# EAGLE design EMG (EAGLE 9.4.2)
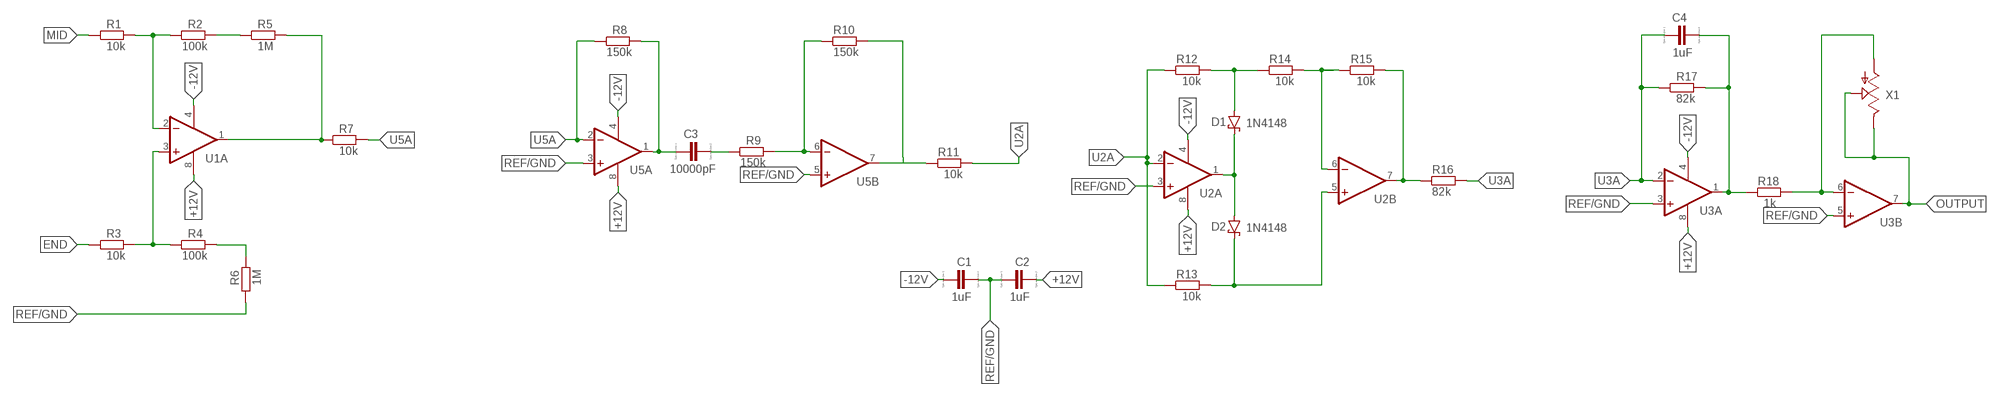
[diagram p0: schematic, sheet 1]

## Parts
C1  1uF  SURFACEMOUNTCC1310  [C1310]
C2  1uF  SURFACEMOUNTCC1310  [C1310]
C3  10000pF  SURFACEMOUNTCC1310  [C1310]
C4  1uF  SURFACEMOUNTCC1310  [C1310]
D1  1N4148  SURFACEMOUNTDIODE  [SOD323_ST]
D2  1N4148  SURFACEMOUNTDIODE  [SOD323_ST]
R1  10k  RESISTORSM0805  [SURFACEMOUNT]
R2  100k  RESISTORSM0805  [SURFACEMOUNT]
R3  10k  RESISTORSM0805  [SURFACEMOUNT]
R4  100k  RESISTORSM0805  [SURFACEMOUNT]
R5  1M  RESISTORSM0805  [SURFACEMOUNT]
R6  1M  RESISTORSM0805  [SURFACEMOUNT]
R7  10k  RESISTORSM0805  [SURFACEMOUNT]
R8  150k  RESISTORSM0805  [SURFACEMOUNT]
R9  150k  RESISTORSM0805  [SURFACEMOUNT]
R10  150k  RESISTORSM0805  [SURFACEMOUNT]
R11  10k  RESISTORSM0805  [SURFACEMOUNT]
R12  10k  RESISTORSM0805  [SURFACEMOUNT]
R13  10k  RESISTORSM0805  [SURFACEMOUNT]
R14  10k  RESISTORSM0805  [SURFACEMOUNT]
R15  10k  RESISTORSM0805  [SURFACEMOUNT]
R16  82k  RESISTORSM0805  [SURFACEMOUNT]
R17  82k  RESISTORSM0805  [SURFACEMOUNT]
R18  1k  RESISTORSM0805  [SURFACEMOUNT]
U1  OPAMPSUA  [SOIC8]
U2  OPAMPSUA  [SOIC8]
U3  OPAMPSUA  [SOIC8]
U5  OPAMPSUA  [SOIC8]
X1  POTENTIOMETERS3223G  [SURFACEMOUNTPOT]

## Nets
+12V: C2.2 U1.8(P:V+) U2.8(P:V+) U3.8(P:V+) U5.8(P:V+)
-12V: C1.1 U1.4(P:V-) U2.4(P:V-) U3.4(P:V-) U5.4(P:V-)
END: R3.1
MID: R1.1
N$1: R1.2 R2.1 U1.2(A:-IN)
N$2: R3.2 R4.1 U1.3(A:+IN)
N$3: R2.2 R5.1
N$4: R4.2 R6.2
N$5: R15.2 R16.1 U2.7(B:OUT)
N$6: C3.1 R8.2 U5.1(A:OUT)
N$7: C3.2 R9.1
N$8: R9.2 R10.1 U5.6(B:-IN)
N$9: R18.2 U3.6(B:-IN) X1.1(A)
N$10: R14.2 R15.1 U2.6(B:-IN)
N$11: D1.C D2.A U2.1(A:OUT)
N$12: D1.A R12.2 R14.1
N$13: D2.C R13.2 U2.5(B:+IN)
N$14: C4.2 R17.2 R18.1 U3.1(A:OUT)
N$15: R10.2 R11.1 U5.7(B:OUT)
N$17: R5.2 R7.1 U1.1(A:OUT)
OUTPUT: U3.7(B:OUT) X1.2(S) X1.3(E)
REF/GND: C1.2 C2.1 R6.1 U2.3(A:+IN) U3.3(A:+IN) U3.5(B:+IN) U5.3(A:+IN) U5.5(B:+IN)
U2A: R11.2 R12.1 R13.1 U2.2(A:-IN)
U3A: C4.1 R16.2 R17.1 U3.2(A:-IN)
U5A: R7.2 R8.1 U5.2(A:-IN)
Unconnected: U1.5(B:+IN) U1.6(B:-IN) U1.7(B:OUT)

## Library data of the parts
C1-C4 = Customized:SURFACEMOUNTC: CAPACITOR, European symbol; SPICEMODEL: NONE; SPICEPREFIX: C
D1 D2 = Customized:SURFACEMOUNTDIODE: Schottky barrier diode
R1-R18 = Customized:RESISTORS: RESISTOR, European symbol; SPICEPREFIX: R
U1-U3 U5 = Customized:OPAMPS: 12V, 7MHz, CMOS, Rail-to-Rail I/O Dual OP AMP Source: http://focus.ti.com/lit/ds/sbos201/sbos201.pdf
X1 = Customized:POTENTIOMETERS: POTENTIOMETER

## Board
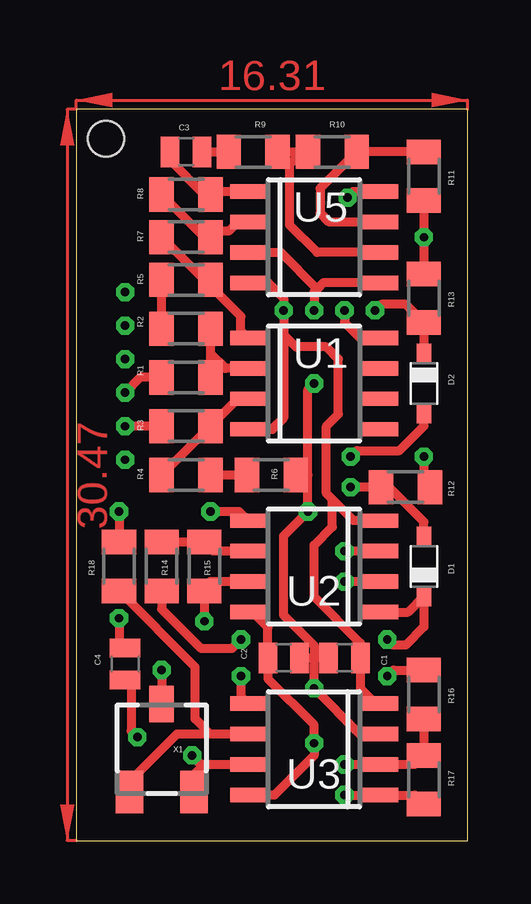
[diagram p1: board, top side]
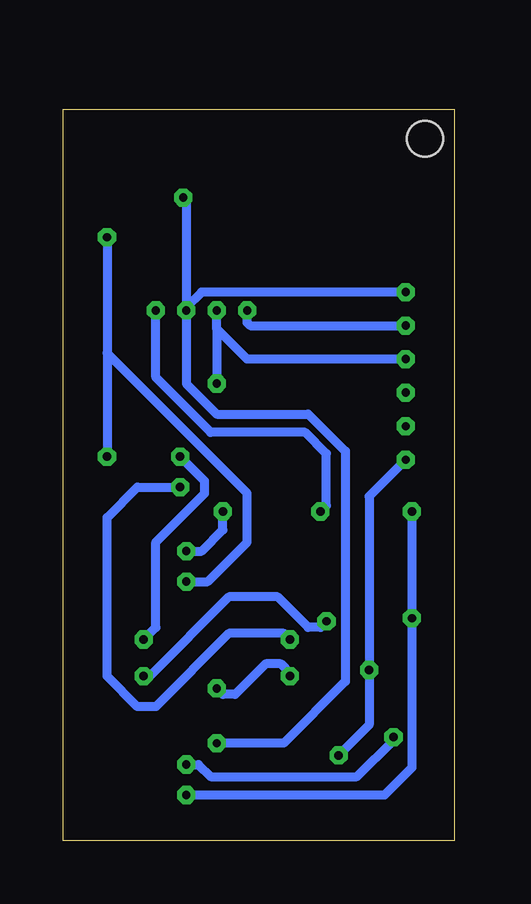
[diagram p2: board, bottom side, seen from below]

Size 16.31 x 30.47 mm. Coordinates in mm from the lower left corner, seen from the top.
Outline: 0,0 16.31,0 16.31,30.47 0,30.47 0,0
Copper layers (1*16): Top 0.035mm / dielectric 1.5mm / Bottom 0.035mm
Design rules "default": minimum track width 6mil, minimum drill 0.35mm, track to track 6mil, track to pad 6mil, pad to pad 6mil, via to via 6mil, smd to smd 6mil, copper to edge 40mil, drill to drill 6mil, minimum pad ring 10mil, minimum via ring 8mil, stop-mask expansion 4mil, vias tented up to drill 0mil, thermal gap 10mil
Holes 1.5 mm at 1.23,29.25

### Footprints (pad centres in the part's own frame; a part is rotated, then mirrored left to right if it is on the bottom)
C1310 = smd 0.771 x 1.27: 1 -0.66,0; 2 0.66,0
SOD323_ST = smd 0.8 x 0.6: A 1.25,0; C -1.25,0
SURFACEMOUNT = smd 1.016 x 1.422: 1 -1.016,0; 2 1.016,0
SOIC8 = smd 0.6 x 1.5: 1 -1.905,-2.75; 2 -0.635,-2.75; 3 0.635,-2.75; 4 1.905,-2.75; 5 1.905,2.75; 6 0.635,2.75; 7 -0.635,2.75; 8 -1.905,2.75
SURFACEMOUNTPOT = smd 1.143 x 1.778: 1 -1.346,-1.778; 3 1.346,-1.778 | smd 1.016 x 1.524: 2 0,1.88

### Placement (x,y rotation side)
C1  11.18,7.62 180 top
C2  8.64,7.62 180 top
C3  4.57,28.7 0 top
C4  2.03,7.37 90 top
D1  14.48,11.43 90 top
D2  14.48,19.05 270 top
R1  4.57,19.3 0 top
R2  4.57,21.34 180 top
R3  4.57,17.27 0 top
R4  4.57,15.24 0 top
R5  4.57,23.37 0 top
R6  8.13,15.24 180 top
R7  4.57,25.15 0 top
R8  4.57,26.92 0 top
R9  7.37,28.7 0 top
R10  10.67,28.7 0 top
R11  14.48,27.69 270 top
R12  13.72,14.73 180 top
R13  14.48,22.61 270 top
R14  3.56,11.43 90 top
R15  5.33,11.43 270 top
R16  14.48,6.1 270 top
R17  14.48,2.54 270 top
R18  1.78,11.43 270 top
U1  9.91,19.05 270 top
U2  9.91,11.43 90 top
U3  9.91,3.81 90 top
U5  9.91,25.15 270 top
X1  3.56,3.81 0 top

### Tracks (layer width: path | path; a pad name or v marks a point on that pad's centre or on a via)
+12V  (via drill 0.35 pad 0.38)
  Top 0.381: U1.8 11.81,20.95 11.18,21.59 v11.18,22.1 | U2.8 7.34,9.53 7.98,8.89 C2.2 7.98,6.76 9.91,4.83 v9.91,4.06 9.91,3.56 8.26,1.91 U3.8 | U5.8 11.56,27.05 v11.3,26.8
  Bottom 0.381: v2.03,22.86 10.54,22.86 11.18,22.23 | v11.3,26.8 11.18,26.67 11.18,22.23 | v9.91,4.06 7.12,4.06 4.55,6.64 4.55,16.23 6.1,17.78 9.91,17.78 11.18,19.05 v11.18,22.1 11.18,22.23
-12V  (via drill 0.35 pad 0.38)
  Top 0.381: U1.4 8.17,17.14 8.64,17.61 8.64,21.08 | U3.4 12.47,5.71 11.84,6.35 C1.1 11.84,8.23 9.91,10.16 9.91,12.32 10.67,13.08 10.67,14.22 | U5.4 8,23.24 8.64,22.61 v8.64,22.1 8.64,21.08 | 8.64,21.08 9.14,20.57 10.41,20.57 10.92,20.07 10.92,17.78 10.41,17.27 10.41,14.48 10.67,14.22 | U2.4 11.56,13.34 10.67,14.22
  Bottom 0.381: v8.64,22.1 8.64,21.59 8.51,21.46 v2.03,21.46
END  (via drill 0.35 pad 0.38)
  Top 0.381: R3.1 v2.03,17.27
MID  (via drill 0.35 pad 0.38)
  Top 0.381: R1.1 2.67,19.3 v2.03,18.67
N$1
  Top 0.381: 5.97,19.68 U1.2 6.22,19.68 5.59,20.32 | R2.1 5.59,20.32 | 5.59,20.32 R1.2
N$2
  Top 0.381: U1.3 6.73,18.41 R3.2 R4.1
N$3
  Top 0.381: R2.2 R5.1
N$4
  Top 0.381: R4.2 R6.2
N$5  (via drill 0.35 pad 0.38)
  Top 0.381: v5.33,9.14 R15.2 5.33,10.54 5.59,10.79 U2.7 | R16.1 13.21,7.11 v12.95,6.86
  Bottom 0.381: v12.95,6.86 12.7,6.86 9.4,10.16 7.37,10.16 6.1,8.89 5.59,8.89 v5.33,9.14
N$6
  Top 0.381: 7.09,27.05 U5.1 5.71,27.05 R8.2 5.33,26.92 3.91,28.35 C3.1
N$7
  Top 0.381: C3.2 R9.1
N$8
  Top 0.381: 8.64,28.7 R9.2 9.4,28.7 | 9.4,28.7 R10.1 | U5.6 10.03,24.51 8.89,25.65 8.89,28.19 9.4,28.7
N$9
  Top 0.381: X1.1 2.21,2.46 4.19,4.45 U3.6 5.59,4.45 4.95,5.08 4.95,7.24 R18.2
N$10
  Top 0.381: 3.58,12.72 R14.2 R15.1 5.71,12.06 U2.6
N$11  (via drill 0.35, 0.35 pad 0.33)
  Top 0.381: 11.61,16.18 v11.43,16 11.68,16.26 13.46,16.26 14.48,17.27 D2.A | 12.91,9.53 U2.1 13.82,9.53 D1.C 14.48,8.91 13.72,8.15 13.19,8.15 v12.95,8.38
  Bottom 0.381: v11.43,16 10.41,14.99 10.41,14.48 12.45,12.45 12.45,8.89 v12.95,8.38
N$12  (via drill 0.35 pad 0.33, 0.35 pad 0.38)
  Top 0.381: 6.83,8.38 v6.86,8.38 6.48,8 5.21,8 3.56,9.65 R14.1 | R12.2 12.7,14.88 | R12.2 v11.43,14.73 | 13.03,14.73 R12.2 | 12.79,14.73 R12.2 | D1.A 14.48,13.28 13.03,14.73 R12.2
  Bottom 0.381: v11.43,14.73 13.21,14.73 14.48,13.46 14.48,6.86 13.21,5.59 12.45,5.59 9.4,8.64 7.11,8.64 v6.86,8.38
N$13  (via drill 0.35, 0.35 pad 0.38)
  Top 0.381: U2.5 6.78,13.72 v5.59,13.72 | v12.45,22.1 12.7,22.35 13.72,22.35 R13.2 D2.C
  Bottom 0.381: v12.45,22.1 12.45,19.3 10.16,17.02 6.22,17.02 5.33,16.13 5.33,13.97 v5.59,13.72
N$14  (via drill 0.35, 0.35 pad 0.33)
  Top 0.381: U3.1 13.08,1.91 | v1.78,13.72 R18.1 | v11.18,1.91 U3.1 | U3.1 14.1,1.91 R17.2 | v1.78,9.27 1.78,8.28 C4.2
  Bottom 0.381: v1.78,13.72 v1.78,9.27 1.78,3.05 2.92,1.91 v11.18,1.91
N$15
  Top 0.381: 14.22,28.7 R11.1 R10.2 10.16,27.18 10.16,26.16 10.54,25.78 U5.7
N$17
  Top 0.381: 5.33,23.37 R7.1 | 5.33,23.37 R5.2 5.59,23.11 | U1.1 6.86,21.25 6.86,21.84 5.33,23.37
OUTPUT  (via drill 0.35, 0.35 pad 0.38)
  Top 0.381: v3.56,7.11 X1.2 | U3.7 5.33,3.17 | 5.33,3.17 5.21,3.17 v4.83,3.56 | X1.3 4.9,2.74 5.33,3.17
  Bottom 0.381: v2.03,15.88 3.56,14.35 v3.56,7.11 3.56,4.83 v4.83,3.56
REF/GND  (via drill 0.35, 0.35 pad 0.33, 0.35 pad 0.38)
  Top 0.381: C2.1 9.93,7.62 | C1.2 9.93,7.62 | 9.93,7.62 9.93,8.1 8.64,9.4 8.64,12.7 v9.65,13.72 9.65,15.24 | 12.57,12.06 U2.3 v11.18,12.06 | U3.5 6.86,6.01 v6.86,6.86 | v9.91,19.05 9.65,18.8 9.65,15.24 | R6.1 9.65,15.24 | U5.3 8.51,24.51 10.03,22.99 | v9.91,22.1 9.91,22.86 10.03,22.99 | U5.5 10.29,23.24 10.03,22.99 | 9.93,7.62 9.91,7.59 v9.91,6.35 11.81,4.45 U3.3
  Bottom 0.381: v11.18,12.06 10.54,12.06 9.65,12.95 v9.65,13.72 | 9.91,21.34 v9.91,19.05 | 9.91,21.34 8.64,20.07 v2.03,20.07 | 9.91,21.34 v9.91,22.1 | v6.86,6.86 6.86,6.99 7.24,7.37 7.87,7.37 9.14,6.1 9.65,6.1 v9.91,6.35
U2A  (via drill 0.35 pad 0.33)
  Top 0.381: 13.08,10.79 U2.2 v11.18,10.79 | v14.48,16 14.48,14.99 R12.1 | R11.2 v14.48,25.15 R13.1
  Bottom 0.381: 14.48,20.32 v14.48,16 | v11.18,10.79 10.29,10.79 8.64,12.45 8.64,14.48 14.48,20.32 | v14.48,25.15 14.48,20.32
U3A  (via drill 0.35 pad 0.33)
  Top 0.381: 13.08,3.17 U3.2 | U3.2 12.68,3.2 | R16.2 R17.1 14.1,3.17 U3.2 | U3.2 v11.18,3.17 | v2.54,4.32 2.29,4.57 2.29,6.45 C4.1
  Bottom 0.381: v11.18,3.17 10.67,3.17 10.16,2.67 4.06,2.67 2.54,4.19 v2.54,4.32
U5A
  Top 0.381: R8.1 5.33,25.15 R7.2 5.84,25.4 6.35,25.4 6.73,25.78 U5.2
(copper drawn outside any net)
  shapes: Top area x2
